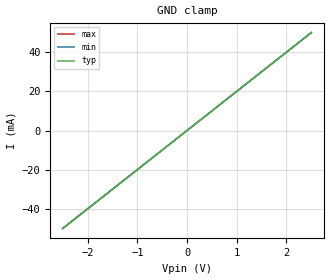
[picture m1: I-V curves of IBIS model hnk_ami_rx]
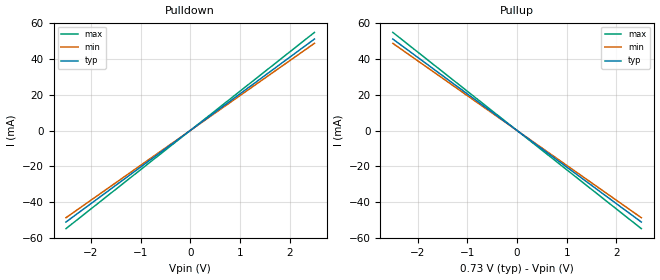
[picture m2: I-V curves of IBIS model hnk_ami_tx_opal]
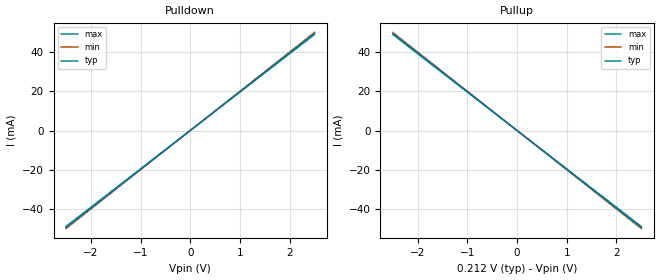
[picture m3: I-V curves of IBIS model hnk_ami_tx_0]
|Copyright 2011 Hank, Inc.
|  Hank, Inc.
[IBIS Ver]   5.0
[Disclaimer] THESE IBIS MODELS ARE PROVIDED FOR TRAING PURPOSES.
[File Name]   hnk_serdes.ibs
[File Rev]   1.0
[Date]   07/22/2012
[Source]   Developed by:
Hank, Inc.
Box 443
West Park, N.Y.
[Notes]
[Copyright] Copyright 2010, Hank, Inc.,
All Rights Reserved.
[Component] hnk_serdes
[Manufacturer] Hank
[Package]
R_pkg   .001   NA   NA
L_pkg   1p   NA   NA
C_pkg   1f   NA   NA
[Pin]   signal_name   model_name   R_pin L_pin  C_pin
1p   hnk_tx_p   hnk_ami_tx   NA   NA   NA
1n   hnk_tx_n   hnk_ami_tx   NA   NA   NA
2p   hnk_rx_p   hnk_ami_rx   NA   NA   NA
2n   hnk_rx_n   hnk_ami_rx   NA   NA   NA
[Diff_Pin] inv_pin vdiff tdelay_typ tdelay_min tdelay_max
1p   1n   0.1V  NA   NA   NA
2p   2n   0.1V  NA   NA   NA
[Model Selector] hnk_ami_tx
hnk_ami_tx_0 0
hnk_ami_tx_opal opal
hnk_ami_tx_1 1
hnk_ami_tx_2 2
| Models and submodels in the file (5): hnk_ami_rx (Input), hnk_ami_tx_opal (Output), hnk_ami_tx_0 (Output), hnk_ami_tx_1 (Output), hnk_ami_tx_2 (Output)
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[Model] hnk_ami_rx
Model_type Input
C_comp 1.769p 1.73p 1.816p
Vinh = 0.55
Vinl = 0.45
[Algorithmic Model]
Executable Windows_VisualStudio7.1.3088_64 hnkdfe2.dll hnkdfe.ami
Executable Linux_gcc3.2.3_64 hnkdfe2.linux.so hnkdfe.ami
[End Algorithmic Model]
[Temperature_Range] 25 100 0
[Voltage Range] 1.0 0.9 1.1
[GND Clamp]
-2.5V     -49.99mA   -49.77mA   -49.9mA
0V        0A         0A         0A
2.5V      49.99mA    49.77mA    49.9mA
[Model] hnk_ami_tx_opal
Model_type Output
C_comp 0.80p 0.75p 0.85p
Cref = 0
Vref = 0.5
Rref = 50
Vmeas = 0.3
[Algorithmic Model]
Executable Windows_VisualStudio7.1.3088_64 hnkffe.dll hnkffe.ami
Executable Linux_gcc3.2.3_64 hnkffe.linux.so hnkffe.ami
[End Algorithmic Model]
[Temperature_Range] 25 100 0
[Voltage Range] 0.73 0.13 1.07
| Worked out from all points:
|   slope of the pulldown table from 0 to 0.11 V, typ, clamps not added: 48.9 ohm
|   slope of the pullup table from 0 to 0.11 V, typ, clamps not added: 48.9 ohm
[Pulldown]
-2.5V     -51.1mA    -48.7mA    -54.8mA
0V        0A         0A         0A
2.5V      51.1mA     48.7mA     54.8mA
[Pullup]
-2.5V     51.1mA     48.7mA     54.8mA
0V        0A         0A         0A
2.5V      -51.1mA    -48.7mA    -54.8mA
[Ramp]
| variable   typ   min   max
dV/dt_r   0.438/1p   0.078/1p   0.642/1p
dV/dt_f   0.438/1p   0.078/1p   0.642/1p
R_load = 50.0000
|   model   hnk_ami_tx_0
[Model] hnk_ami_tx_0
Model_type Output
C_comp 800f 750f 850f
Cref = 0
[Model Spec]
Vmeas .106 .101 .111
Vref .106 .101 .111
[Temperature Range]  25 100 0
[Voltage Range] .212 .202 .221
[Algorithmic Model]
Executable Windows_VisualStudio7.1.3088_64 hnkffe.dll hnkffe.ami
Executable Linux_gcc3.2.3_64 hnkffe.linux.so hnkffe.ami
[End Algorithmic Model]
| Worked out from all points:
|   slope of the pulldown table from 0 to 0.032 V, typ, clamps not added: 50.7 ohm
|   slope of the pullup table from 0 to 0.032 V, typ, clamps not added: 50.7 ohm
[Pulldown]
-2.5V     -49.36mA   -49.91mA   -48.82mA
0V        0A         0A         0A
2.5V      49.36mA    49.91mA    48.82mA
[Pullup]
-2.5V     49.36mA    49.91mA    48.82mA
0V        0A         0A         0A
2.5V      -49.36mA   -49.91mA   -48.82mA
[Ramp]
|dV/dt_r .063/60f .061/60f .066/60f
|dV/dt_f .063/60f .061/60f .066/60f
dV/dt_r 63/60p 61/60p 66/60p
dV/dt_f 63/60p 61/60p 66/60p
